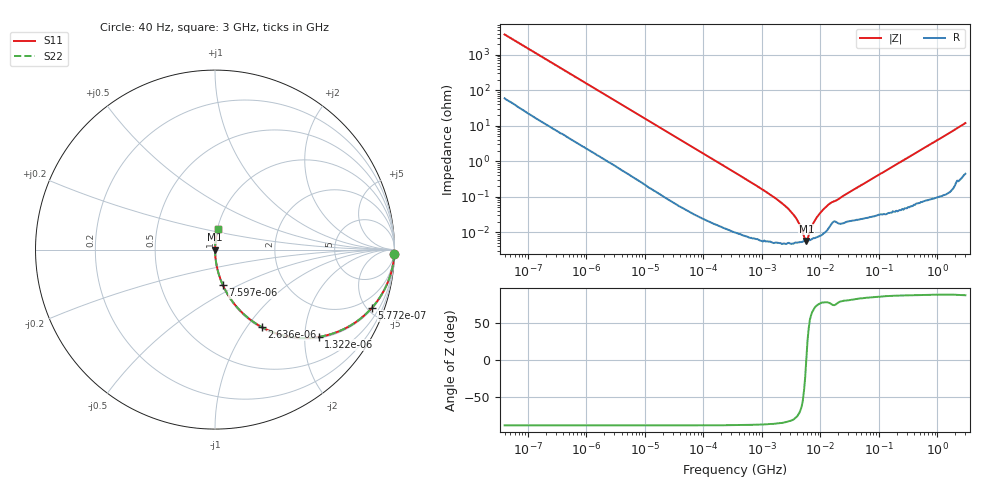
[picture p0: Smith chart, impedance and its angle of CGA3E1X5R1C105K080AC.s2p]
! S-parameter Generated by TDK Corporation
! Copyright(C) 2015 TDK Corporation.
! All Rights Reserved.
! TDK P/N: CGA3E1X5R1C105K080AC (Multilayer Ceramic Chip Capacitors)
! Property: C=1uF
! Size(LxWxT): 1.6x0.8x0.8mm, 0.063x0.031x0.031inches
! Model Type: s2p (Touchstone File Format Version 1.0)
! Frequency: DC=Yes Start=0.00004MHz Stop=3000MHz 396points Log-sweep
! Note: This model was converted from impedance.
! Model Generated on Jun. 23, 2015
! Hash(MD5):
! Port Assignments:
!  1 ---| |--- 2
! Applicable Conditions:
!  Temperature = 25 degC
!  DC Bias Voltage = 0 V
!  Small Signal Operation
! Terms and conditions regarding TDK Simulation Models
! (1)This simulation model is being provided solely for informational purposes. Please refer to the specifications of the products in terms of detailed characteristics of such products.
! (2)In no event shall TDK Corporation of any of its subsidiaries be liable for any loss or damage arising, directly or indirectly,
!  From any information contained in this simulation model, including, but not limited to loss or damages arising from any inaccuracies, omissions or errors in connection with such information.
! (3)Any and all copyrights on this simulation model are owned by TDK Corporation.
!  Duplication or redistribution of this simulation model without prior written permission from TDK Corporation is prohibited.
! (4)This simulation model is subject to any modification or change without any prior notice.
! (5)Neither TDK Corporation nor any of its subsidiaries shall make any warranty, express or implied,
!  Including but not limited to the correctness, implied warranties of merchantability and fitness for a particular purpose with respect to this simulation models.
! (6)The use of this simulation model shall be deemed to have consented to the terms and conditions hereof.
# MHz S MA R 50
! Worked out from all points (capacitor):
!   395 points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, 40 Hz to 3 GHz, reference 50 ohm
!   read as one part in series: C = 1.06 uF near 41.88 Hz
!   lowest |Z| = 5.72 mohm at 5.739 MHz (marker M1)
!   series resonance near 5.719 MHz, so ESL is about 730 pH
!   S11 on the Smith chart (normalised r, x): 40 Hz: 2, -75; 577.2 Hz: 1.08, -5.33; 1.322 kHz: 1.03, -2.35; 2.636 kHz: 1.02, -1.18; 7.597 kHz: 1.01, -0.42; 3 GHz: 1.01, +0.24
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4e-05  0.9992 -1.5  0.0266 87.6  0.0266 87.6  0.9992 -1.5
0.0001826612  0.9912 -6.8  0.1186 82.4  0.1186 82.4  0.9912 -6.8
0.0005772088  0.9318 -20.4  0.3494 68.7  0.3494 68.7  0.9318 -20.4
0.000834128  0.8745 -28.2  0.4724 61.0  0.4724 61.0  0.8745 -28.2
0.001321622  0.7555 -40.1  0.6441 49.1  0.6441 49.1  0.7555 -40.1
0.002635842  0.506 -58.8  0.8551 30.4  0.8551 30.4  0.506 -58.8
0.00437302  0.3363 -69.5  0.937 19.6  0.937 19.6  0.3363 -69.5
0.007596806  0.2034 -77.5  0.9762 11.7  0.9762 11.7  0.2034 -77.5
0.01739424  0.09186 -84.0  0.9946 5.3  0.9946 5.3  0.09186 -84.0
0.3464102  0.00481 -88.6  0.9999 0.3  0.9999 0.3  0.00481 -88.6
1.094655  0.001487 -87.7  0.9999 0.1  0.9999 0.1  0.001487 -87.7
2.286002  0.0006232 -85.6  1 0.0  1 0.0  0.0006232 -85.6
3.792615  0.0002562 -78.4  0.9999 0.0  0.9999 0.0  0.0002562 -78.4
4.998775  9.542e-05 -55.2  0.9999 0.0  0.9999 0.0  9.542e-05 -55.2
5.738865  5.716e-05 2.1  0.9999 -0.0  0.9999 -0.0  5.716e-05 2.1
6.588528  0.0001017 54.3  0.9999 -0.0  0.9999 -0.0  0.0001017 54.3
7.22376  0.0001524 65.0  0.9999 -0.0  0.9999 -0.0  0.0001524 65.0
9.521122  0.0003218 76.1  0.9999 -0.0  0.9999 -0.0  0.0003218 76.1
14.40706  0.0006404 77.2  0.9999 -0.0  0.9999 -0.0  0.0006404 77.2
150.6385  0.006214 86.4  0.9996 -0.4  0.9996 -0.4  0.006214 86.4
994.0817  0.03933 86.3  0.9983 -2.3  0.9983 -2.3  0.03933 86.3
3000  0.1183 81.1  0.9886 -6.8  0.9886 -6.8  0.1183 81.1
